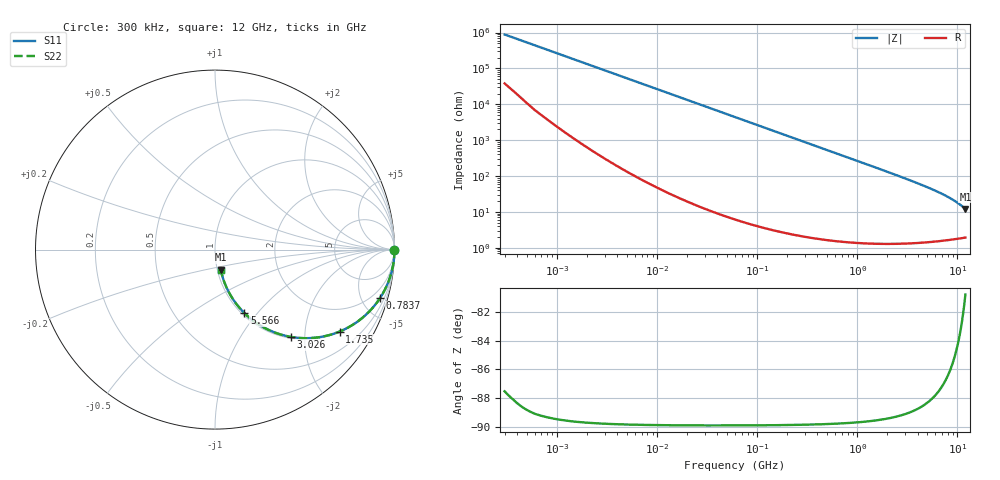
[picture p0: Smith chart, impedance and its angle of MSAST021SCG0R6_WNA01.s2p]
! MSAST021SCG0R6_WNA01  S-PARAMETER MODEL  ( General Type )
! Model Generated by TAIYO YUDEN Corporation (http://www.ty-top.com)
! Version 2.0
! TAIYO YUDEN Control No. 181101
! Copyright(c) 2015 TAIYO YUDEN CO.,LTD. All Rights Reserved.
! Product Description (link to TY-COMPAS)
! https://ds.yuden.co.jp/TYCOMPAS/or/detail?pn=MSAST021SCG0R6BWNA01&u=M
! Products Name : Multilayer Ceramic Capacitors
! Characteristics :
!  Capacitance : 0.6 pF , Rated Voltage : 25V , TCC : CG / C0G
!  Case Size : 0.25 x 0.125 / 0.0098 x 0.0049 [mm/inch] , Thickness : 0.125 / 0.0049 [mm/inch]
!  (Conditions: Temperature = 25 degC , DC Bias Current/Voltage = 0A / 0V)
! External Node Assignments :
!  1  o---| |---o  2
! GND o---------o GND
! Frequency Range : 0.3MHz  -  12000MHz  [ 401 STEP ]
# MHz S RI R 50
! Freq[MHz].  S11 Real  S11 Imag  S21 Real  S21 Imag  S12 Real  S12 Imag  S22 Real  S22 Imag
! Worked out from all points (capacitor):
!   401 points, 300 kHz to 12 GHz, reference 50 ohm
!   read as one part in series: C = 600 fF near 316.3 kHz
!   lowest |Z| = 12 ohm at 12 GHz (marker M1)
!   S11 on the Smith chart (normalised r, x): 300 kHz: open; 783.7 MHz: 1.03, -6.76; 1.735 GHz: 1.03, -3.03; 3.026 GHz: 1.03, -1.70; 5.566 GHz: 1.03, -0.86; 12 GHz: 1.04, -0.24
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0.3  1 -0.000113  4.87e-06 0.000113  4.87e-06 0.000113  1 -0.000113
0.316324  1 -0.000119  4.78e-06 0.000119  4.78e-06 0.000119  1 -0.000119
1.769972  1 -0.000667  3.94e-06 0.000667  3.94e-06 0.000667  1 -0.000667
10.44266  1 -0.00394  2.24e-05 0.00394  2.24e-05 0.00394  1 -0.00394
60  0.9995 -0.0226  0.000543 0.0226  0.000543 0.0226  0.9995 -0.0226
164.1901  0.9961 -0.0617  0.00392 0.0617  0.00392 0.0617  0.9961 -0.0617
353.9943  0.9822 -0.1311  0.0178 0.1311  0.0178 0.1311  0.9822 -0.1311
555.3718  0.9573 -0.2005  0.0427 0.2005  0.0427 0.2005  0.9573 -0.2005
783.7017  0.9185 -0.2716  0.0815 0.2716  0.0815 0.2716  0.9185 -0.2716
1166.079  0.8354 -0.3679  0.1646 0.3679  0.1646 0.3679  0.8354 -0.3679
1403.667  0.7775 -0.4125  0.2225 0.4125  0.2225 0.4125  0.7775 -0.4125
1735.023  0.6947 -0.4563  0.3053 0.4563  0.3053 0.4563  0.6947 -0.4563
2088.533  0.6095 -0.4828  0.3905 0.4828  0.3905 0.4828  0.6095 -0.4828
2514.07  0.5163 -0.4935  0.4837 0.4935  0.4837 0.4935  0.5163 -0.4935
3026.31  0.421 -0.4861  0.579 0.4861  0.579 0.4861  0.421 -0.4861
3944.255  0.2938 -0.445  0.7062 0.445  0.7062 0.445  0.2938 -0.445
5565.855  0.1638 -0.3535  0.8362 0.3535  0.8362 0.3535  0.1638 -0.3535
7064.448  0.1018 -0.2785  0.8982 0.2785  0.8982 0.2785  0.1018 -0.2785
8503.825  0.0679 -0.2192  0.9321 0.2192  0.9321 0.2192  0.0679 -0.2192
9968.853  0.0474 -0.1691  0.9526 0.1691  0.9526 0.1691  0.0474 -0.1691
11380.75  0.0355 -0.1283  0.9645 0.1283  0.9645 0.1283  0.0355 -0.1283
12000  0.0319 -0.1123  0.9681 0.1123  0.9681 0.1123  0.0319 -0.1123
